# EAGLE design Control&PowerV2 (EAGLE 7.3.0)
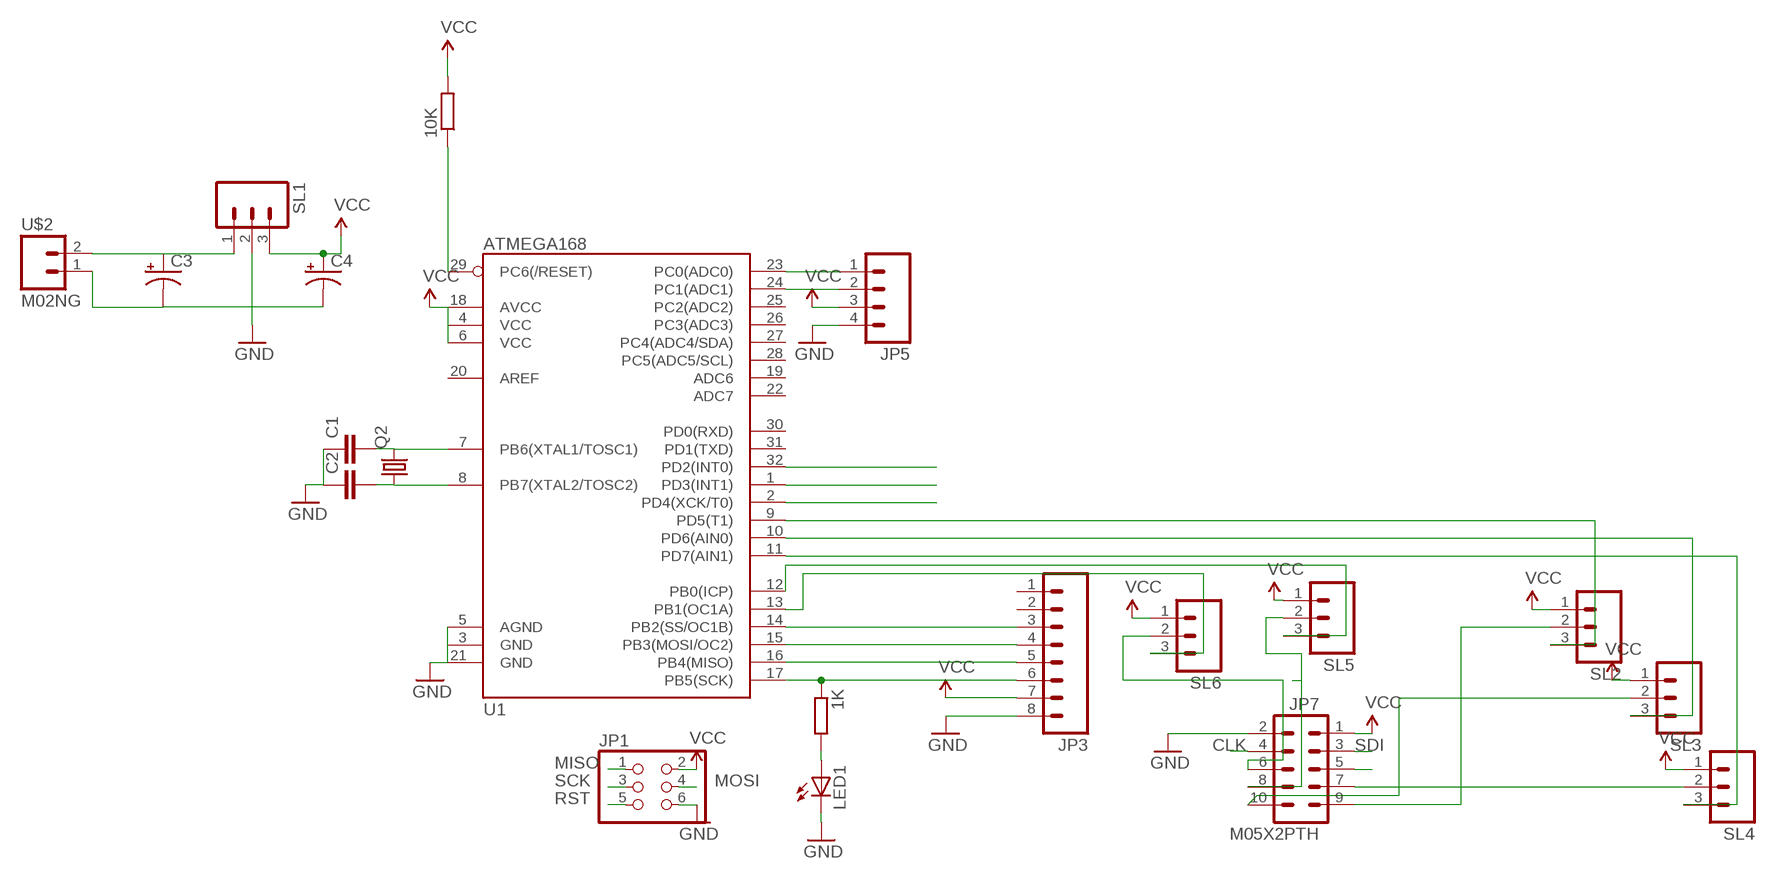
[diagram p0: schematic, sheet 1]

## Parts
1K  R-EU_0207/10  [0207/10]
10K  R-EU_0207/10  [0207/10]
C1  C5/3.5  [C5B3.5]
C2  C5/3.5  [C5B3.5]
C3  CAP_POLPTH1  [CPOL-RADIAL-100UF-25V]
C4  CAP_POLPTH1  [CPOL-RADIAL-100UF-25V]
JP1  PINHD-2X3  [2X03]
JP3  M08  [1X08]
JP5  M04LONGPADS  [1X04_LONGPADS]
JP7  M05X2PTH  [AVR_ICSP]
LED1  LED5MM  [LED5MM]
Q2  CRYSTALHC18U-V  [HC18U-V]
SL1  M03  [03P]
SL2  M03  [03P]
SL3  M03  [03P]
SL4  M03  [03P]
SL5  M03  [03P]
SL6  M03  [03P]
U1  ATMEGA168  [TQFP32-08]
U$2  M02NG  [1X02]

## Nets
CLK: JP7.4 U1.1(PD3(INT1))
GND: C1.1 C2.1 C3.2(-) C4.2(-) JP1.6 JP3.8 JP5.4 JP7.2 LED1.K(C) SL1.2 U1.3(GND) U1.5(AGND) U1.21(GND) U$2.1
LE: JP7.5 U1.2(PD4(XCK/T0))
MISO: JP1.1 JP3.5 U1.16(PB4(MISO))
MOSI: JP1.4 JP3.4 U1.15(PB3(MOSI/OC2))
N$1: C1.2 Q2.2 U1.7(PB6(XTAL1/TOSC1))
N$2: C2.2 Q2.1 U1.8(PB7(XTAL2/TOSC2))
N$3: SL2.3 U1.9(PD5(T1))
N$4: C3.1(+) SL1.1 U$2.2
N$5: JP3.3 U1.14(PB2(SS/OC1B))
N$6: JP5.1 U1.23(PC0(ADC0))
N$7: JP5.2 U1.24(PC1(ADC1))
N$9: JP7.10 SL3.2
N$10: SL3.3 U1.10(PD6(AIN0))
N$11: SL4.3 U1.11(PD7(AIN1))
N$15: SL5.3 U1.12(PB0(ICP))
N$17: SL6.3 U1.13(PB1(OC1A))
N$18: JP7.9 SL2.2
N$19: 1K.2 LED1.A
N$21: JP7.7 SL4.2
N$22: JP7.8 SL5.2
N$23: JP7.6 SL6.2
RST: 10K.1 JP1.5 U1.29(PC6(/RESET))
SCK: 1K.1 JP1.3 JP3.6 U1.17(PB5(SCK))
SDI: JP7.3 U1.32(PD2(INT0))
VCC: 10K.2 C4.1(+) JP1.2 JP3.7 JP5.3 JP7.1 SL1.3 SL2.1 SL3.1 SL4.1 SL5.1 SL6.1 U1.4(VCC) U1.6(VCC) U1.18(AVCC)
Unconnected: JP3.1 JP3.2 U1.19(ADC6) U1.20(AREF) U1.22(ADC7) U1.25(PC2(ADC2)) U1.26(PC3(ADC3)) U1.27(PC4(ADC4/SDA)) U1.28(PC5(ADC5/SCL)) U1.30(PD0(RXD)) U1.31(PD1(TXD))

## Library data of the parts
1K 10K = resistor:R-EU_: RESISTOR, European symbol
C1 C2 = capacitor-wima:C: CAPACITOR
C3 C4 = SparkFun:CAP_POL: Capacitor Polarized
JP1 = SparkFun:PINHD-2X3: PIN HEADER
JP3 = SparkFun:M08: Header 8 Standard 8-pin 0.1" header. Use with straight break away headers (SKU : PRT-00116), right angle break away headers (PRT-00553), swiss pins (PRT-00743), machine pins (PRT-00117), and female headers (PRT-00115).
JP5 = SparkFun:M04: Header 4 Standard 4-pin 0.1" header. Use with straight break away headers (SKU : PRT-00116), right angle break away headers (PRT-00553), swiss pins (PRT-00743), machine pins (PRT-00117), and female headers (PRT-00115). Molex polarized connector foot print use with SKU : PRT-08231 with associated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
JP7 = SparkFun:M05X2: Header 5x2 Standard 10-pin dual row 0.1" header. Commonly used with AVR-ISP. Use with Spark Fun Electronics SKU: PRT-00778
LED1 = led:LED: LED
Q2 = crystal:CRYSTAL: CRYSTAL; OC_FARNELL: unknown; OC_NEWARK: unknown
SL1-SL6 = con-amp-quick:M03: AMP QUICK CONNECTOR; OC_FARNELL: unknown; OC_NEWARK: unknown
U1 = SparkFun:ATMEGA168
U$2 = SparkFun:M02NG

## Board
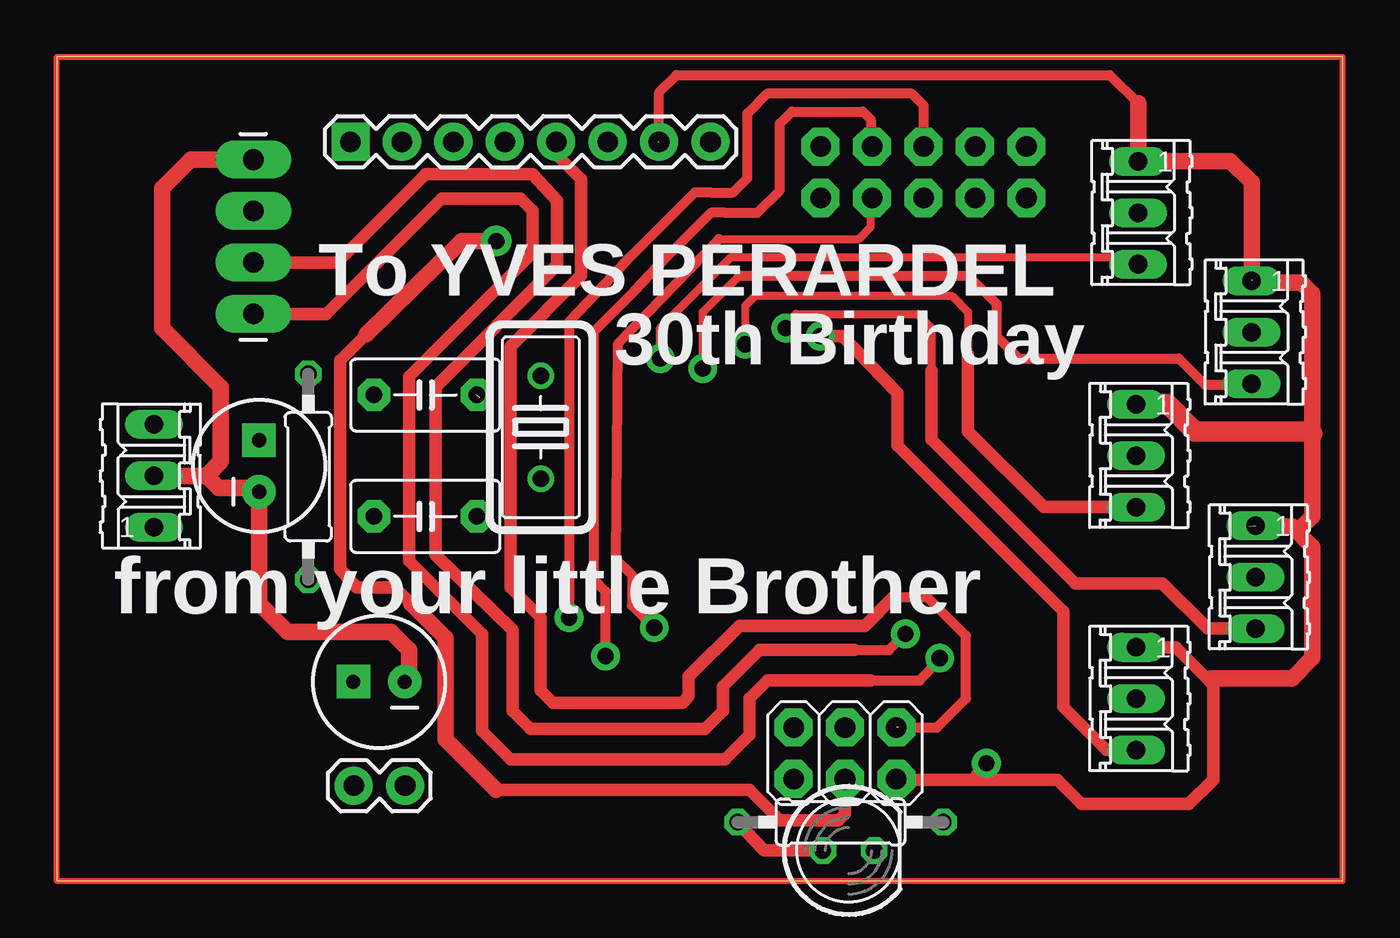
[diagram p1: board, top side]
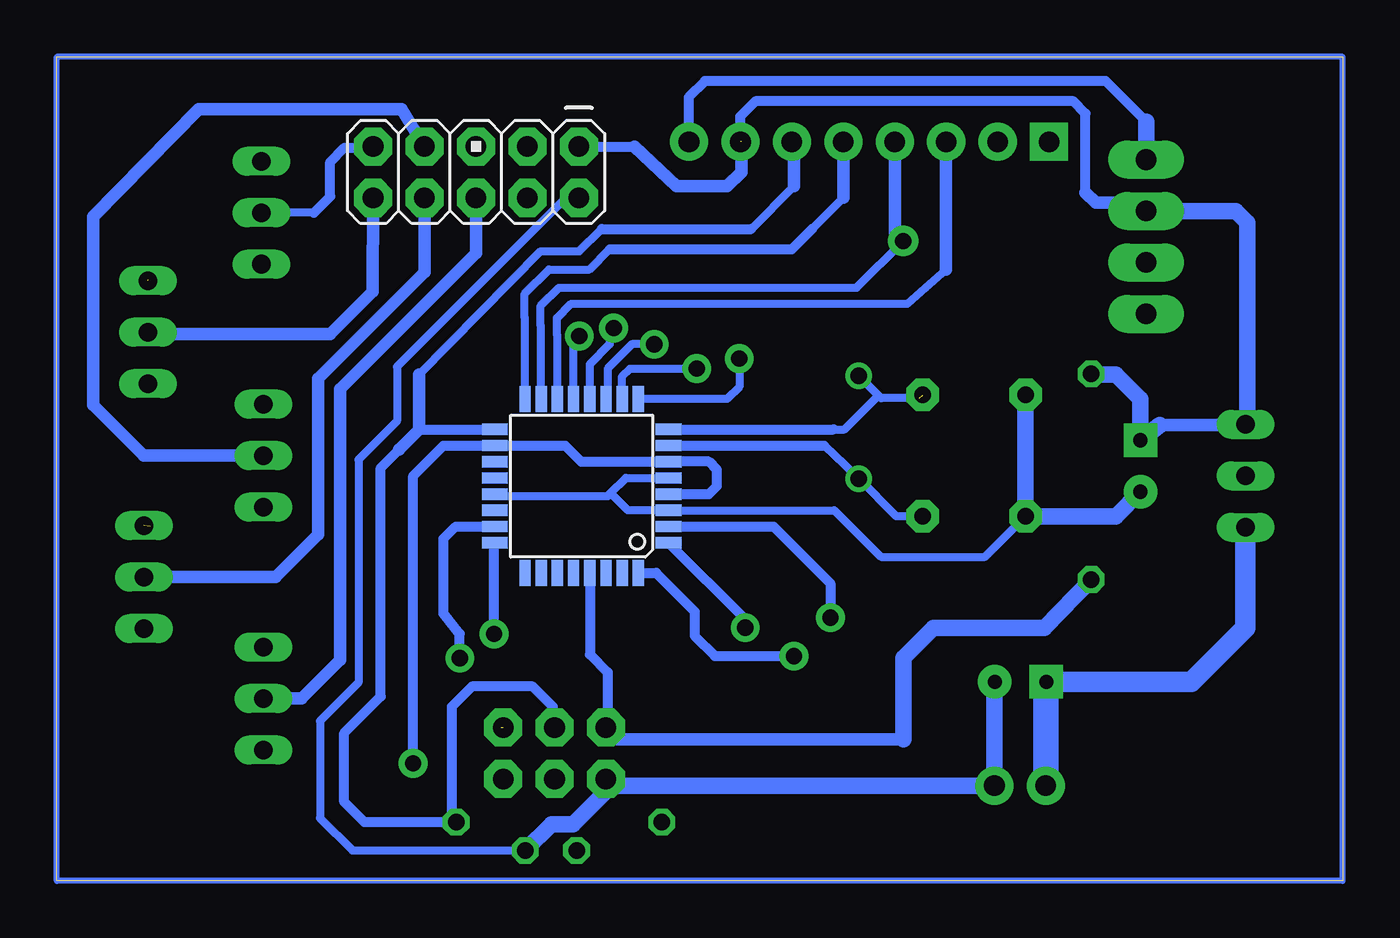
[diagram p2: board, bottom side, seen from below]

Size 63.5 x 40.7 mm. Coordinates in mm from the lower left corner, seen from the top.
Outline: 0,0 63.5,0 63.5,40.7 0,40.7 0,0
Copper layers (1*16): Top 0.035mm / dielectric 1.5mm / Bottom 0.035mm
Design rules "default": minimum track width 10mil, minimum drill 24mil, track to track 8mil, track to pad 8mil, pad to pad 8mil, via to via 8mil, smd to smd 8mil, copper to edge 40mil, drill to drill 8mil, minimum pad ring 10mil, minimum via ring 8mil, stop-mask expansion 4mil, vias tented up to drill 0mil, thermal gap 10mil

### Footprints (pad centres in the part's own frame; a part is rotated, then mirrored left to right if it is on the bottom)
0207/10 = drill 0.813 octagon: 1 -5.08,0; 2 5.08,0
C5B3.5 = drill 0.813 pad 1.6 octagon: 1 -2.54,0; 2 2.54,0
CPOL-RADIAL-100UF-25V = drill 0.7 pad 1.651 square: 1 1.27,0 | drill 0.7 pad 1.651: 2 -1.27,0
2X03 = drill 1.016 pad 1.88 octagon: 1 -2.54,-1.27; 2 -2.54,1.27; 3 0,-1.27; 4 0,1.27; 5 2.54,-1.27; 6 2.54,1.27
1X08 = drill 1.016 pad 1.88 square: 1 0,0 | drill 1.016 pad 1.88: 2 2.54,0; 3 5.08,0; 4 7.62,0; 5 10.16,0; 6 12.7,0; 7 15.24,0; 8 17.78,0
1X04_LONGPADS = drill 1.016 pad 1.88 long: 1 0,0; 2 2.54,0; 3 5.08,0; 4 7.62,0
AVR_ICSP = drill 1.016 pad 1.88 octagon: 1 -1.27,5.08; 2 1.27,5.08; 3 -1.27,2.54; 4 1.27,2.54; 5 -1.27,0; 6 1.27,0; 7 -1.27,-2.54; 8 1.27,-2.54; 9 -1.27,-5.08; 10 1.27,-5.08
LED5MM = drill 0.813 octagon: A -1.27,0; K 1.27,0
HC18U-V = drill 0.813: 1 -2.54,0; 2 2.54,0
03P = drill 0.914 long: 1 -2.54,0; 2 0,0; 3 2.54,0
TQFP32-08 = smd 1.27 x 0.559: 1 -4.293,2.8; 2 -4.293,2; 3 -4.293,1.2; 4 -4.293,0.4; 5 -4.293,-0.4; 6 -4.293,-1.2; 7 -4.293,-2; 8 -4.293,-2.8; 17 4.293,-2.8; 18 4.293,-2; 19 4.293,-1.2; 20 4.293,-0.4; 21 4.293,0.4; 22 4.293,1.2; 23 4.293,2; 24 4.293,2.8 | smd 0.559 x 1.27: 9 -2.8,-4.293; 10 -2,-4.293; 11 -1.2,-4.293; 12 -0.4,-4.293; 13 0.4,-4.293; 14 1.2,-4.293; 15 2,-4.293; 16 2.8,-4.293; 25 2.8,4.293; 26 2,4.293; 27 1.2,4.293; 28 0.4,4.293; 29 -0.4,4.293; 30 -1.2,4.293; 31 -2,4.293; 32 -2.8,4.293
1X02 = drill 1.016 pad 1.88: 1 0,0; 2 2.54,0

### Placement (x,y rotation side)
1K  38.7,2.9 180 top
10K  12.42,19.96 90 top
C1  18.2,18 0 top
C2  18.2,24 0 top
C3  15.91,9.83 180 top
C4  9.99,20.49 90 top
JP1  38.92,6.3 180 top
JP3  14.5,36.5 0 top
JP5  9.7,28 90 top
JP7  42.8,35 270 bottom
LED1  39.1,1.5 0 top
Q2  23.9,22.4 270 top
SL1  4.8,20 90 top
SL2  53.4,33 270 top
SL3  59,27.1 270 top
SL4  53.3,21 270 top
SL5  59.2,15 270 top
SL6  53.3,9 270 top
U1  37.58,19.5 180 bottom
U$2  17.2,4.7 180 top

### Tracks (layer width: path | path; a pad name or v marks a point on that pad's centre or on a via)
CLK  (via drill 0.8 pad 1.42)
  Top 0.406: 32.7,31.7 39.6,31.7 40.2,32.3 40.2,33.67 JP7.4
  Top 0.5: 32.7,31.7 27.7,26.5 27.6,15.9 28.4,15.1 28.4,13.6 v29.5,12.5
  Bottom 0.4: v29.5,12.5 29.5,12.91
  Bottom 0.5: 29.5,12.91 U1.1
GND
  Top 0.813: SL1.2 7.4,20 | 7.4,20 8,19.4 9.81,19.4 C4.2 9.99,13.71 11.4,12.3 16.5,12.3 17.4,11.4 17.4,10.05 C3.2 | JP5.4 6.62,35.62 5.2,34.2 5.2,27.3 8.1,24.4 8.1,20.7 7.4,20
  Bottom 0.406: JP7.2 38.37,33.73 46.7,25.4 46.7,22.7 48.6,20.8 48.6,9.8 50.5,7.9 50.5,3.1 48.9,1.5 LED1.K | U1.21 41.5,19.1 41.4,19 36.3,19 36.15,19.15 | 36.15,19.15 35.4,19.9 U1.5 | C1.1 17.66,16 22.8,16 25.1,18.3 U1.3 35.3,18.3 36.15,19.15
  Bottom 0.5: 9.7,37.5 11.7,39.5 31.5,39.5 32.3,38.7 32.3,36.52
  Bottom 0.61: 32.3,36.52 JP3.8
  Bottom 0.813: JP1.6 36.38,4.5 | 36.38,4.5 36.38,4.42 38,2.8 39.07,2.8 LED1.K | C4.2 11.21,18 C1.1 C2.1 | 9.7,37.5 JP5.4 | 36.38,4.5 36.18,4.7 U$2.1 17.2,9.81 C3.2
LE  (via drill 0.8 pad 1.42)
  Top 0.5: v25.3,13 25.3,27.6 27.1,29.5 28.3,30.8 31.5,34 32.3,34 33.4,34 34.1,34.7 34.1,37.9 35.1,38.9 42.2,38.9 42.8,38.3 42.8,36.3 43.2,35.9 43.17,35.9 JP7.5
  Bottom 0.5: U1.2 28.1,17.5 25.3,14.7 v25.3,13
MISO  (1 unrouted)
  Top 0.5: 41.57,7.57 43.47,7.57 44.9,9 44.9,12.1 43,14 41.3,14
  Top 0.61: JP3.5 24.66,35.9 25.9,34.66 25.9,29.9 22.4,26.4 22.4,14.5 23.9,13 23.9,9.4 24.5,8.8 30.9,8.8 31.2,9.1 31.2,10.1 33.7,12.6 39.9,12.6 41.3,14
  Bottom 0.4: 24.66,33.74 26.2,32.2 | 40.4,27.8 40.4,23.81
  Bottom 0.406: 40.4,27.8 40.4,29 39.2,30.2 37.2,30.2 36.2,31.2
  Bottom 0.5: 40.4,23.81 U1.16 | 36.2,31.2 27.2,31.2 26.2,32.2
  Bottom 0.61: JP3.5 24.66,33.74
MOSI  (via drill 0.8 pad 1.5)
  Top 0.61: JP1.4 38.92,3.32 38.6,3 35.7,3 34.2,4.5 21.7,4.5 | 17.5,13.7 16.7,14.5 14.8,14.5 14,15.4 14,25.7 15.3,27
  Top 0.813: 21.7,4.5 19.2,7 19.2,12 17.5,13.7 | 15.3,27 20,31.6 v21.7,31.6
  Bottom 0.4: 39.6,27.4 39.6,23.81
  Bottom 0.406: 39.6,23.87 U1.15 | 39.6,27.4 39.6,28.4 38.7,29.3 24,29.3 v21.7,31.6
  Bottom 0.5: 39.6,23.81 U1.15
  Bottom 0.61: JP3.4 22.12,32.02 v21.7,31.6
N$1
  Bottom 0.406: C1.2 22.04,18 Q2.2 24.6,20.56 25.6,21.5
  Bottom 0.5: U1.7 25.6,21.5
N$2  (1 unrouted)
  Bottom 0.406: 20.9,23.84 22.8,23.84 22.93,23.97 | 22.93,23.97 Q2.1 | 25.14,22.3 24.6,22.3 22.93,23.97
  Bottom 0.5: U1.8 25.14,22.3
N$3  (via drill 0.8 pad 1.42)
  Top 0.406: v29.8,25.8 29.8,27.3 33.3,30.8 52.6,30.8 53.4,30.5 53.31,30.5 53.31,30.46 SL2.3
  Bottom 0.4: v29.8,25.8 29.8,24.4 30.4,23.8 U1.9
N$4
  Bottom 0.61: SL1.1 4.8,17.39
  Bottom 0.813: C3.1 14.66,9.31
  Bottom 1.016: C3.1 7.47,9.83 4.8,12.5 4.8,17.39
  Bottom 1.27: 14.66,9.31 U$2.2
N$5
  Bottom 0.4: 38.8,27 38.8,23.81
  Bottom 0.406: 38.8,24.17 U1.14 | 19.6,30.2 20.6,29.3 21.5,28.5 38.1,28.5 38.8,27.8 38.8,27 | 19.6,36.48 JP3.3
  Bottom 0.5: 38.8,23.81 U1.14
  Bottom 0.61: 19.6,30.2 19.6,36.48
N$6  (via drill 0.8 pad 1.42)
  Top 0.5: 40.2,9.9 42.6,9.9 43.1,10.4 43.3,10.7 v43.6,11
  Top 0.61: JP5.1 13.3,28 19,33.7 22.9,33.7 23.5,33.1 23.5,31 17.4,24.9 17.4,15.8 21,12.2 21,7.4 22.4,6 33,6 34.2,7.2 34.2,9 35.1,9.9 40.2,9.9
  Bottom 0.5: v43.6,11 43.6,12.2 44.4,13.2 44.4,16.9 43.8,17.5 U1.23
N$7  (via drill 0.8 pad 1.42)
  Top 0.5: 39.4,11.4 41.1,11.4 v41.9,12.2
  Top 0.61: JP5.2 13.84,30.54 18.2,34.9 23.5,34.9 24.7,33.6 24.7,30.4 18.7,24.4 18.7,16.1 22.5,12.4 22.5,8.4 23.4,7.5 32,7.5 32.9,8.4 32.9,9.6 34.7,11.4 39.4,11.4
  Bottom 0.5: v41.9,12.2 41.9,16.67 U1.24
N$9
  Bottom 0.61: JP7.10 47.9,29.11 50,27 59,27 SL3.2
N$10  (via drill 0.8 pad 1.42)
  Top 0.406: v31.9,25.3 31.9,28.1 33.7,29.9
  Top 0.5: 33.7,29.9 45,29.9 46.4,28.5 46.4,26.9 47.5,25.8 55.4,25.8 56.7,24.5 58.81,24.5
  Top 0.813: SL3.3 58.81,24.56 58.81,24.5
  Bottom 0.4: U1.10 35.58,24.92 35.2,25.3 v31.9,25.3
N$11  (via drill 0.8 pad 1.42)
  Top 0.406: v34,26.5 34,28.4 34.5,28.9 44.2,28.9 45,28.1 45,26
  Top 0.61: 45,26 45,22.2 48.74,18.46 SL4.3
  Bottom 0.4: v34,26.5 35.1,26.5 36.3,25.3 36.3,23.87 U1.11
N$13
  Bottom 0.305: 0,0 0,40.7 63.5,40.7 63.5,0 0,0
N$14
  Top 0.305: 0,40.7 63.5,40.7 63.5,0 0,0 0,40.7
N$15  (via drill 0.8 pad 1.42)
  Top 0.406: v36,27.3 36.2,27.7 36.5,28 42.5,28 43.2,27.3 43.2,25.2
  Top 0.61: 43.2,25.2 43.2,21.8 50.3,14.7 54.6,14.7 56.84,12.46 SL5.3
  Bottom 0.406: U1.12 37.18,25.52 36.2,26.5 v36,27.3
N$17  (via drill 0.8 pad 1.42)
  Top 0.61: v37.7,26.9 38.8,26.9 41.5,24.1 41.5,21.5 49.7,13.3 49.7,8.6 51.84,6.46 SL6.3
  Bottom 0.4: U1.13 37.98,26.52 v37.7,26.9
N$18
  Bottom 0.406: 50.8,33 SL2.2
  Bottom 0.5: 50.8,33 50,33.8 50,35.5 49.3,36.2 47.95,36.2 JP7.9
N$19
  Top 0.61: LED1.A 34.92,1.5 1K.2
N$21
  Bottom 0.61: JP7.7 46.47,38.1 56.5,38.1 61.7,32.8 61.7,23.5 59.2,21 SL4.2
N$22
  Bottom 0.61: JP7.8 45.34,30.06 50.6,24.8 50.6,17.1 52.7,15 SL5.2
N$23
  Bottom 0.61: JP7.6 42.8,31 49.5,24.3 49.5,10.9 51.4,9 SL6.2
RST
  Bottom 0.5: U1.29 37.18,11.18 36.3,10.3 36.3,7.65 JP1.5
  Bottom 0.61: 21.7,7 35.81,7 JP1.5
  Bottom 0.813: 10K.1 14.74,12.5 20.2,12.5 21.7,11 21.7,7
SCK
  Bottom 0.4: 29.2,32.2 27.1,34.3 | 39.6,31.1 45.6,25
  Bottom 0.406: 39.6,31.1 37.7,31.1 36.6,32.2
  Bottom 0.5: 45.6,22.3 U1.17 | 1K.1 44.3,2.9 | 44.3,2.9 48.3,2.9 49.3,3.9 49.3,7.3 47.5,9.1 47.5,20.4 46.6,21.3 | JP1.3 38.92,7.82 39,7.9 39,8.6 40,9.6 43,9.6 44,8.6 44,3.2 44.3,2.9 | 36.6,32.2 29.2,32.2
  Bottom 0.61: 27.1,34.3 27.1,36.4 JP3.6 | 46.6,21.3 45.6,22.3 45.6,25
SDI  (via drill 0.8 pad 1.42)
  Top 0.5: v27.1,11.1 27.1,14.3 26.5,14.9 26.5,27.1 28.5,29.1 30.1,30.8 32.3,33 33,33 34.6,33 35.7,34.1 35.7,37.4 36.3,38 39.8,38 40.2,37.6 40.2,36.33 JP7.3
  Bottom 0.5: U1.32 33.91,15.21 32,13.3 32,12.1 31,11.1 v27.1,11.1
VCC  (via drill 0.8 pad 1.42)  (3 unrouted)
  Top 0.406: 61,17.5 61.5,17.5 | SL2.1 53.4,35.59
  Top 0.5: 45.4,5 45.4,5.3 v45.9,5.8 | JP3.7 29.74,38.94 30.6,39.8 52,39.8 53.4,38.4
  Top 0.61: 56.95,9.85 55.26,11.54 SL6.1 | 56.95,9.85 57.1,9.7 57.1,5 55.9,3.8 50.6,3.8 49.4,5 45.4,5 41.49,5 JP1.2 | 57,10 57,9.9 56.95,9.85
  Top 0.813: 59,29.69 59,34.5 57.96,35.54 SL2.1 | 61.5,17.5 62,18 62,22.1 62,29 61.46,29.54 59,29.54 SL3.1 | 58.89,17.5 61,17.5 62,16.5 62,11 61,10 57,10 | 53.4,38.4 53.4,35.59
  Top 1.016: SL4.1 54.86,23.54 56.2,22.2 61.9,22.2 62,22.1
  Bottom 0.406: 12.36,25 10K.2 | JP5.3 10.12,33.5
  Bottom 0.5: 12.7,34 12.7,37.9 13.3,38.5 29,38.5 29.74,37.76 JP3.7 | JP7.1 34.97,36.27 | U1.4 31.3,19.1 30.9,19.5 30.9,20.3 31.3,20.7 U1.6 37.6,20.7 38.4,21.5 U1.18 44.4,21.5 45.9,20 v45.9,5.8
  Bottom 0.61: 12.7,34 12.2,33.5 10.12,33.5 | 34.97,36.27 32.9,34.3 30.4,34.3 29.7,35 29.7,36.5 | 9.03,22.52 4.82,22.52 SL1.3 4.78,22.52 4.7,22.52
  Bottom 0.813: 9.03,22.52 C4.1 9.99,23.79 11.2,25 12.36,25 | JP5.3 5.28,33.08 4.7,32.5 4.7,22.52

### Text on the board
tPlace: To YVES PERARDEL | 30th Birthday | from your little Brother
